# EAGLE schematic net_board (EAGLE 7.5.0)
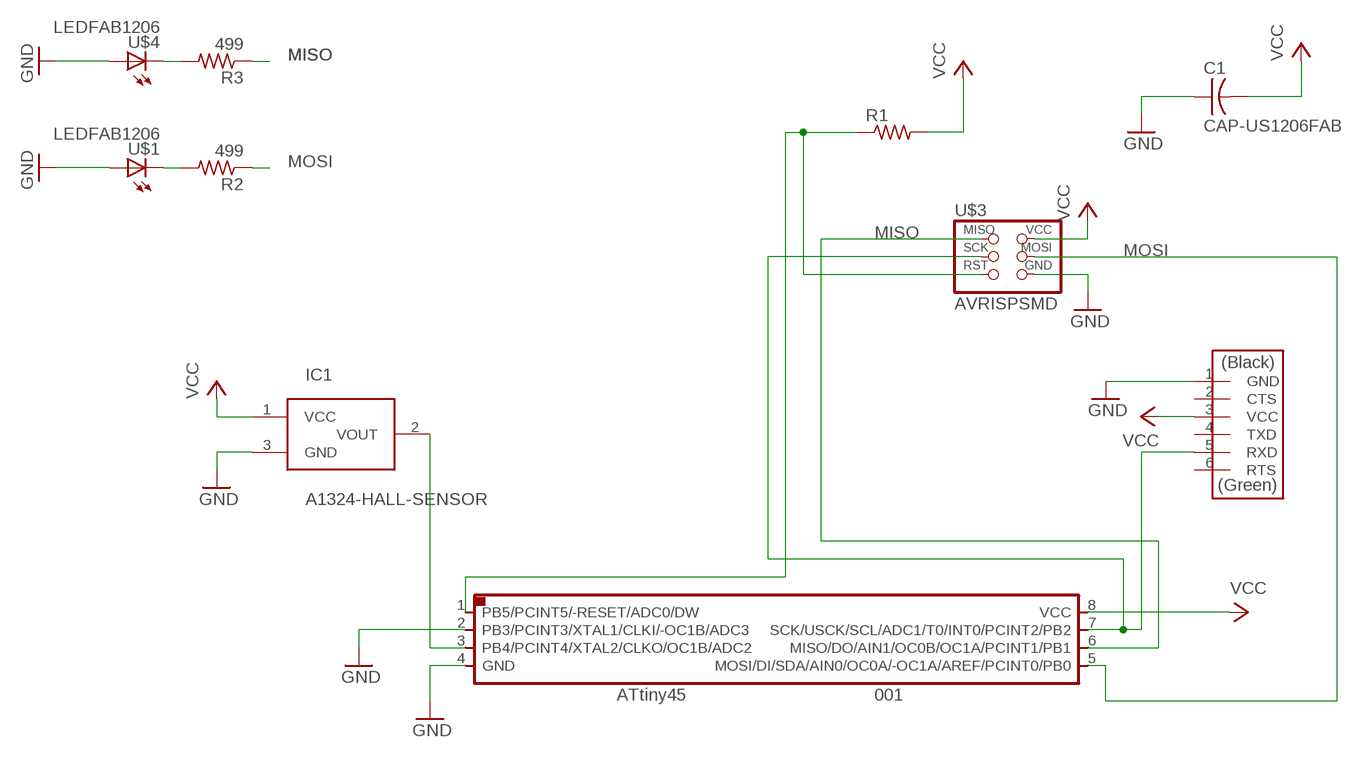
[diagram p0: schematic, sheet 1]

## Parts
001  ATTINY45SI  [SOIC8]
C1  CAP-US1206FAB  [C1206FAB]
IC1  A1324-HALL-SENSOR  [SOT23]
R1  RES-US1206FAB  [R1206FAB]
R2  499  RES-US1206FAB  [R1206FAB]
R3  499  RES-US1206FAB  [R1206FAB]
U$1  LEDFAB1206  [LED1206FAB]
U$2  FTDI-SMD-HEADER  [1X06SMD]
U$3  AVRISPSMD  [2X03SMD]
U$4  LEDFAB1206  [LED1206FAB]

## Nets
GND: 001.2(PB3/PCINT3/XTAL1/CLKI/-OC1B/ADC3) 001.4(GND) C1.1 IC1.3(GND) U$1.1(A) U$2.1(GND) U$3.6(GND) U$4.1(A)
MISO: 001.6(MISO/DO/AIN1/OC0B/OC1A/PCINT1/PB1) R3.1 U$3.1(MISO)
MOSI: 001.5(MOSI/DI/SDA/AIN0/OC0A/-OC1A/AREF/PCINT0/PB0) R2.1 U$3.4(MOSI)
N$1: 001.7(SCK/USCK/SCL/ADC1/T0/INT0/PCINT2/PB2) U$2.5(RXD) U$3.3(SCK)
N$2: 001.1(PB5/PCINT5/-RESET/ADC0/DW) R1.1 U$3.5(RST)
N$4: 001.3(PB4/PCINT4/XTAL2/CLKO/OC1B/ADC2) IC1.2(VOUT)
N$6: R2.2 U$1.2(C)
N$8: R3.2 U$4.2(C)
VCC: 001.8(VCC) C1.2 IC1.1(VCC) R1.2 U$2.3(VCC) U$3.2(VCC)
Unconnected: U$2.2(CTS) U$2.4(TXD) U$2.6(RTS)

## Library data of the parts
001 = fab:ATTINY45
C1 = fab:CAP-US
IC1 = fab:A1324-HALL-SENSOR
R1 = fab:RES-US: Resistor (US Symbol)
R2 R3 = fablab:RES-US: Resistor (US Symbol)
U$1 U$4 = fablab:LED: LED
U$2 = fab:FTDI-SMD-HEADER
U$3 = fab:AVRISP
